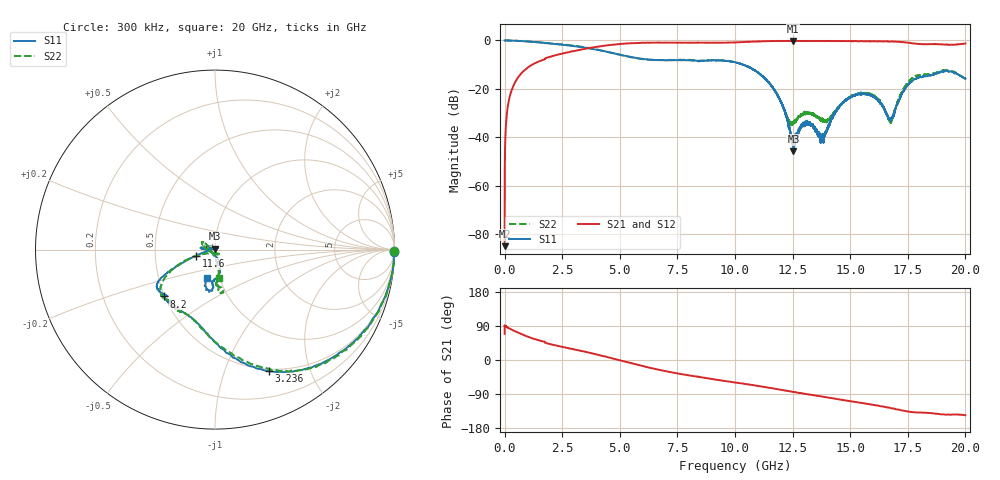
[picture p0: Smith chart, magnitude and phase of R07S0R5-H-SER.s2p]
!{R07S0R5}
!Johanson Technology Inc.
!www.johansontechnology.com
!Test Board Conditions:
!Substrate Type  RO4350B
!Substrate Thickness  10 mil
!Substrate Dk  3.66
!TL Type: GCPW
!TL Trace Width  21 mil
!TL Gap  20 mil
!Electrode orientation  Horizontal
!DUT TOPOLOGY	SERIES
!Mounting Pad LxW  16x21 mil
! Created Fri Feb  5 23:02:59 2021
# hz S ma R 50
! 2 Port Network Data from SP1.SP block
! freq  magS11  angS11  magS21  angS21  magS12  angS12  magS22  angS22
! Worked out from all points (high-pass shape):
!   20001 points, 300 kHz to 20 GHz, reference 50 ohm
!   highest |S21| = -0.17 dB at 12.52 GHz (marker M1); lowest = -85.0 dB at 300 kHz (marker M2)
!   |S21| within 3 dB of the highest: 3.658 GHz to end of sweep
!   lowest |S11| = -45.8 dB at 12.54 GHz (marker M3), VSWR 1.01, Z = 49.9 + j0.494 ohm
!   |S11| at or under -10 dB: 10.34108 GHz to 10.34272 GHz (1.639 MHz wide, 0.0158 % of centre); 10.34 GHz to end of sweep
!   |S22| runs from -35.0 to 0.0 dB; largest |S21 - S12| = 0.011
!   S11 on the Smith chart (normalised r, x): 300 kHz: open; 3.236 GHz: 0.48, -1.43; 8.2 GHz: 0.50, -0.30; 11.6 GHz: 0.81, -0.06; 20 GHz: 0.87, -0.28
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300000  0.9993 -0.6  5.646e-05 69.0  5.52e-05 76.9  0.9991 -0.6
1.303e8  0.9991 -4.0  0.04065 85.7  0.04059 86.0  0.9988 -3.9
4.843e8  0.9848 -14.3  0.1448 75.0  0.1446 75.0  0.9867 -14.2
1.3203e9  0.9237 -34.5  0.3392 55.0  0.3394 54.9  0.9319 -34.0
3.2363e9  0.7398 -66.0  0.6354 25.1  0.6356 25.3  0.7504 -63.2
3.3343e9  0.7304 -67.4  0.6516 23.8  0.6503 23.8  0.7421 -64.7
6.6673e9  0.394 -115.0  0.9039 -25.4  0.9039 -25.3  0.3935 -113.6
8.2003e9  0.385 -137.3  0.8997 -42.6  0.8982 -42.5  0.3934 -125.6
1.00003e10  0.3548 -151.2  0.9123 -59.2  0.914 -59.2  0.3553 -147.3
1.16043e10  0.1111 -161.6  0.9692 -74.6  0.9721 -74.5  0.1118 -161.5
1.20813e10  0.04441 -170.9  0.9746 -79.6  0.9783 -79.6  0.04288 -151.3
1.25213e10  0.005785 104.6  0.9803 -84.3  0.9787 -84.1  0.01989 -81.4
1.25353e10  0.005143 105.5  0.978 -84.4  0.9788 -84.2  0.02014 -75.7
1.29153e10  0.01825 41.1  0.9734 -87.8  0.9749 -88.1  0.02836 -49.6
1.33343e10  0.01801 36.6  0.9741 -92.2  0.976 -92.2  0.0311 -55.7
1.38013e10  0.01141 109.0  0.976 -97.0  0.977 -97.0  0.02324 -97.6
1.45303e10  0.04312 172.9  0.9716 -104.1  0.9704 -104.1  0.04435 178.4
1.54503e10  0.07832 174.1  0.9665 -112.9  0.9655 -112.9  0.0812 151.8
1.61963e10  0.06006 176.1  0.9605 -120.2  0.9602 -120.5  0.06192 148.6
1.66673e10  0.02503 -150.3  0.9494 -125.5  0.9535 -125.8  0.02392 -170.4
1.78033e10  0.1605 -86.1  0.8625 -138.0  0.862 -137.8  0.1791 -86.9
2e10  0.1625 -105.5  0.8647 -145.7  0.863 -145.6  0.1614 -82.2
